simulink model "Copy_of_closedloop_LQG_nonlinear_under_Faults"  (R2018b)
settings: Solver=ode45  StartTime=0.0  StopTime=1500  RelTol=1e-10  AbsTol=1e-10
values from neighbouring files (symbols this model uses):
  Atap = [-atap/A1*sqrt(2*g)    0   0   0    [initial_quadtank_nonlinear.m]
  Dcup = diag([1/A1 1/A2 1/A3 1/A4])    [initial_quadtank_nonlinear.m]
  Qn = eye(size(G,2))*0.01    [initialize_closed_loop_system.m]    (also in Load_Data.m; run_experiment.m = eye(size(G,2))*0)
  Rn = eye(p)*0.0025    [initialize_closed_loop_system.m]    (also in Load_Data.m; run_experiment.m = eye(p)*0)
  sys_tmp = ss(A*1,[B G]*1,C,[D H],Ts)    [initialize_closed_loop_system.m]    (also in Load_Data.m = ss(A,[B Ba],[C; Cp],[D Da; Dp, Dp, zeros(size(Dp,1),ny)],Ts))
  Ts = 2    [initialize_closed_loop_system.m]    (also in Load_Data.m = 0; run_experiment.m = sysmp_d.Ts)
  u0 = [u10;u20]    [initial_quadtank_nonlinear.m]    (also in setup_quadtank_nonlinear.m)
  ub = 25    [msfcn_quadtank_nonlinear.m]    (also in initialize_closed_loop_system.m = 15; Load_Data.m = 15)
  ul = 0    [initialize_closed_loop_system.m]    (also in Load_Data.m)
  x0 = x.^2    [initial_quadtank_nonlinear.m]    (also in setup_quadtank_nonlinear.m)
  y0 = kc*x0(1:2)    [initial_quadtank_nonlinear.m]    (also in setup_quadtank_nonlinear.m)
undefined symbols (not defined in the file or in its folder): An, Bn, Klq
libraries: cstblocks x2

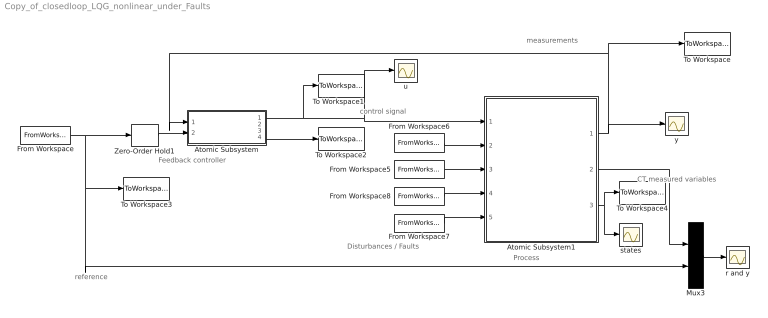
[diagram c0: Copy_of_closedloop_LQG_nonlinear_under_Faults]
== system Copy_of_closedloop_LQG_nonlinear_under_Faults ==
  note: control signal
  note: CT measured variables
  note: reference
  note: measurements
  note: Disturbances / Faults
  note: Process
  note: Feedback controller
  Atomic Subsystem : Subsystem  TreatAsAtomicUnit=on
  Atomic Subsystem1 : Subsystem
  From Workspace : FromWorkspace  VariableName=ref  SampleTime=0  Interpolate=off  OutputAfterFinalValue=Holding final value
  From Workspace5 : FromWorkspace  VariableName=dtap  SampleTime=0  Interpolate=off  OutputAfterFinalValue=Holding final value
  From Workspace6 : FromWorkspace  VariableName=dcup  SampleTime=0  Interpolate=off  OutputAfterFinalValue=Holding final value
  From Workspace7 : FromWorkspace  VariableName=fsensor  SampleTime=0  Interpolate=off  OutputAfterFinalValue=Holding final value
  From Workspace8 : FromWorkspace  VariableName=factuator  SampleTime=0  Interpolate=off  OutputAfterFinalValue=Holding final value
  Mux3 : Mux  Inputs=2
  To Workspace : ToWorkspace  VariableName=measurement  SaveFormat=Timeseries  SampleTime=-1
  To Workspace1 : ToWorkspace  VariableName=control_signal  SaveFormat=Timeseries  SampleTime=-1
  To Workspace2 : ToWorkspace  VariableName=residuals  SaveFormat=Timeseries  SampleTime=-1
  To Workspace3 : ToWorkspace  VariableName=reference  SaveFormat=Timeseries  SampleTime=-1
  To Workspace4 : ToWorkspace  VariableName=state_signals  SaveFormat=Timeseries  SampleTime=-1
  Zero-Order Hold1 : ZeroOrderHold  SampleTime=Ts
  r and y : Scope
  states : Scope
  u : Scope
  y : Scope
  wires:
  From Workspace/1 -> Mux3/2, To Workspace3/1, Zero-Order Hold1/1
  Zero-Order Hold1/1 -> Atomic Subsystem/2(ref)
  Mux3/1 -> r and y/1
  Atomic Subsystem1/1(y_meas) -> Atomic Subsystem/1(y), To Workspace/1, y/1
  Atomic Subsystem/1(u) -> u/1, Atomic Subsystem1/1(u2), To Workspace1/1
  From Workspace6/1 -> Atomic Subsystem1/2(pulse disturbance)
  From Workspace5/1 -> Atomic Subsystem1/3(leakage fault)
  From Workspace8/1 -> Atomic Subsystem1/4(actuator fault)
  From Workspace7/1 -> Atomic Subsystem1/5(sensor fault)
  Atomic Subsystem1/2(y_continuous) -> Mux3/1
  Atomic Subsystem/4(residuals) -> To Workspace2/1
  Atomic Subsystem1/3(x internal) -> states/1, To Workspace4/1

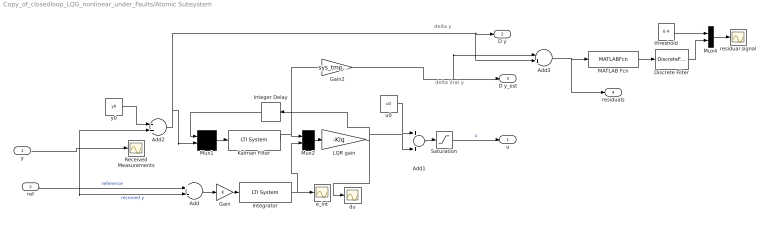
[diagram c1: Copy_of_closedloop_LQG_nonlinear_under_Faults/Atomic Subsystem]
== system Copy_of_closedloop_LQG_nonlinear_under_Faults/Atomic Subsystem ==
  note: delta \hat y
  note: delta y
  y : Inport
  ref : Inport  Port=2
  Add : Sum  Inputs=+-
  Add1 : Sum
  Add2 : Sum  Inputs=-+
  Add3 : Sum  Inputs=-+
  Discrete Filter : DiscreteFilter  Numerator=[0 (1-0.05)]  Denominator=[1 -0.05]  SampleTime=Ts
  Gain : Gain
  Gain2 : Gain  Gain=sys_tmp.c  Multiplication=Matrix(K*u) (u vector)
  Integer Delay : Delay  DelayLength=1  InputProcessing=Inherited
  Integrator : cstblocks/LTI System  sys=sys_int  IC=0
  Kalman Filter : cstblocks/LTI System  sys=F  IC=0
  LQR gain : Gain  Gain=-Klq  Multiplication=Matrix(K*u) (u vector)
  MATLAB Fcn : MATLABFcn  MATLABFcn=norm(u,2)
  Mux1 : Mux  Inputs=2
  Mux2 : Mux  Inputs=2
  Mux4 : Mux  Inputs=2
  Received Measurements : Scope
  Saturation : Saturate  UpperLimit=ub  LowerLimit=ul
  du : Scope
  e_int : Scope
  residual signal : Scope
  threshold : Constant  Value=0.4  VectorParams1D=off
  u0 : Constant  Value=u0  VectorParams1D=off
  y0 : Constant  Value=y0  VectorParams1D=off
  u : Outport
  D y : Outport  Port=2
  D y_est : Outport  Port=3
  residuals : Outport  Port=4
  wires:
  Add2/1 -> Add3/2, D y/1, Mux1/2
  y0/1 -> Add2/1
  Mux2/1 -> LQR gain/1
  Integrator/1 -> Mux2/2, e_int/1
  Mux1/1 -> Kalman Filter/1
  Add1/1 -> Saturation/1
  Add/1 -> Gain/1
  u0/1 -> Add1/1
  ref/1 -> Add/1  "reference"
  LQR gain/1 -> Add1/2, Integer Delay/1, du/1
  Gain/1 -> Integrator/1
  y/1 -> Add/2, Add2/2, Received Measurements/1  "received y"
  Integer Delay/1 -> Mux1/1
  Kalman Filter/1 -> Gain2/1, Mux2/1
  Gain2/1 -> Add3/1, D y_est/1
  Saturation/1 -> u/1  "u"
  Add3/1 -> residuals/1, MATLAB Fcn/1
  Mux4/1 -> residual signal/1
  threshold/1 -> Mux4/1
  MATLAB Fcn/1 -> Discrete Filter/1
  Discrete Filter/1 -> Mux4/2

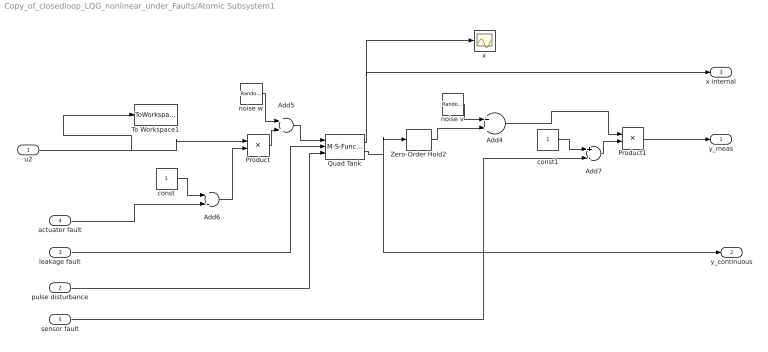
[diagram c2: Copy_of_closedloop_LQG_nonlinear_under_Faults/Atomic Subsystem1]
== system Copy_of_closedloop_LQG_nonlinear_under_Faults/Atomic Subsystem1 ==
  u2 : Inport
  pulse disturbance : Inport  Port=2
  leakage fault : Inport  Port=3
  actuator fault : Inport  Port=4
  sensor fault : Inport  Port=5
  Add4 : Sum
  Add5 : Sum
  Add6 : Sum  Inputs=+-
  Add7 : Sum  Inputs=+-
  Product : Product
  Product1 : Product
  Quad Tank : M-S-Function  FunctionName=msfcn_quadtank_nonlinear  Parameters=x0,An,Bn,Atap,Dcup
  To Workspace1 : ToWorkspace  VariableName=control_signal1  SaveFormat=Timeseries  SampleTime=-1
  Zero-Order Hold2 : ZeroOrderHold  SampleTime=Ts
  const : Constant  VectorParams1D=off
  const1 : Constant  VectorParams1D=off  SampleTime=Ts
  noise v : RandomNumber  Mean=0*diag(Rn)  Variance=diag(Rn)*1  Seed=[0;10]  SampleTime=Ts  VectorParams1D=off
  noise w : RandomNumber  Mean=0*diag(Qn)  Variance=diag(Qn)*1  Seed=[0;20]  SampleTime=Ts  VectorParams1D=off
  x : Scope
  y_meas : Outport
  y_continuous : Outport  Port=2
  x internal : Outport  Port=3
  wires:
  Add5/1 -> Quad Tank/1
  Zero-Order Hold2/1 -> Add4/2
  Quad Tank/1 -> x internal/1, x/1
  noise v/1 -> Add4/1
  noise w/1 -> Add5/1
  Quad Tank/2 -> y_continuous/1, Zero-Order Hold2/1
  Add6/1 -> Product/2
  const/1 -> Add6/1
  Product/1 -> Add5/2
  u2/1 -> To Workspace1/1, Product/1
  const1/1 -> Add7/1
  Add7/1 -> Product1/2
  Add4/1 -> Product1/1
  Product1/1 -> y_meas/1
  pulse disturbance/1 -> Quad Tank/3
  leakage fault/1 -> Quad Tank/2
  actuator fault/1 -> Add6/2
  sensor fault/1 -> Add7/2
